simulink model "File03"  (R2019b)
settings: Solver=FixedStepDiscrete  StartTime=0.0  StopTime=50  FixedStep=1  RelTol=1e-3

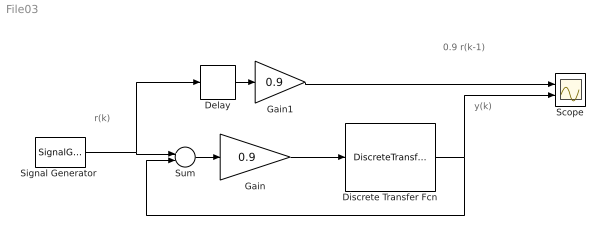
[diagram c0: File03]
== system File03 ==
  note: r(k)
  note: 0.9 r(k-1)
  note: y(k)
  Delay : Delay  DelayLength=1
  Discrete Transfer Fcn : DiscreteTransferFcn  Denominator=[1 -0.9]
  Gain : Gain  Gain=0.9
  Gain1 : Gain  Gain=0.9
  Scope : Scope  NumInputPorts=2
  "Signal Generator " : SignalGenerator  Units=rad/sec
  Sum : Sum  Inputs=+-
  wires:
  Discrete Transfer Fcn/1 -> Scope/2, Sum/2
  "Signal Generator "/1 -> Delay/1, Sum/1
  Sum/1 -> Gain/1
  Gain/1 -> Discrete Transfer Fcn/1
  Delay/1 -> Gain1/1
  Gain1/1 -> Scope/1
